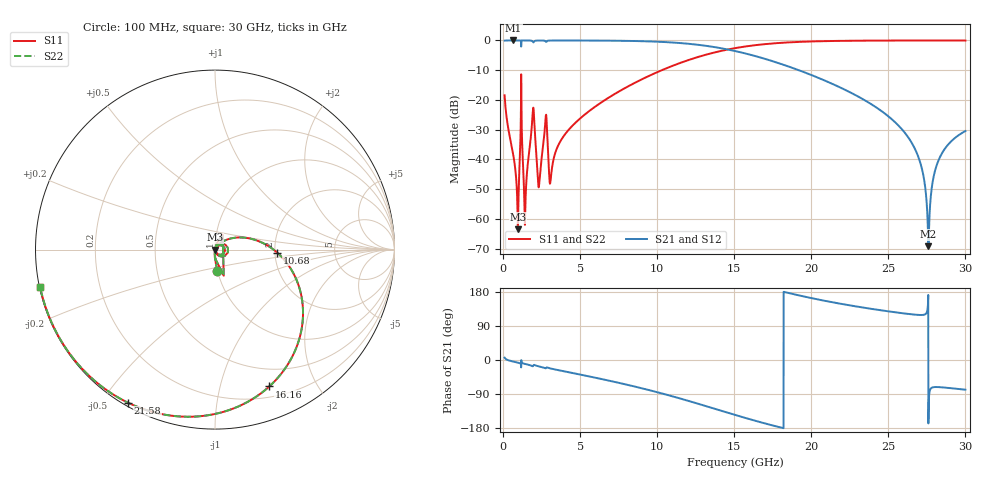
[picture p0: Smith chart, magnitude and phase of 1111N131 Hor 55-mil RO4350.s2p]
# GHz S MA R 50
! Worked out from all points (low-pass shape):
!   3201 points, 100 MHz to 30 GHz, reference 50 ohm
!   highest |S21| = -0.01 dB at 660.6 MHz (marker M1); lowest = -69.2 dB at 27.6 GHz (marker M2)
!   |S21| within 3 dB of the highest: start of sweep to 14.54 GHz
!   lowest |S11| = -63.5 dB at 959.6 MHz (marker M3), VSWR 1.00, Z = 50.1 - j0.0252 ohm
!   |S11| at or under -10 dB: start of sweep to 10.3 GHz
!   |S22| runs from -63.5 to 0.0 dB; largest |S21 - S12| = 0
!   S11 on the Smith chart (normalised r, x): 100 MHz: 1.00, -0.24; 10.68 GHz: 2.06, -0.08; 16.16 GHz: 0.31, -1.43; 21.58 GHz: 0.01, -0.58; 30 GHz: 0.00, -0.10
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0.1  0.1197 -83.7  0.9926 6.1  0.9926 6.1  0.1197 -83.7
0.660625  0.01189 -91.9  0.9994 -4.1  0.9994 -4.1  0.01189 -91.9
0.959625  0.0006712 -22.0  0.9992 -7.0  0.9992 -7.0  0.0006712 -22.0
1.183875  0.1533 -71.5  0.9398 -0.3  0.9398 -0.3  0.1533 -71.5
1.492219  0.003471 63.5  0.9989 -11.0  0.9989 -11.0  0.003471 63.5
1.922031  0.05953 30.9  0.9585 -16.5  0.9585 -16.5  0.05953 30.9
2.333156  0.003607 11.6  0.9966 -17.0  0.9966 -17.0  0.003607 11.6
2.734938  0.04014 35.7  0.9775 -21.7  0.9775 -21.7  0.04014 35.7
3.108687  0.005107 32.5  0.9967 -22.7  0.9967 -22.7  0.005107 32.5
3.697344  0.01972 57.9  0.9979 -27.7  0.9979 -27.7  0.01972 57.9
5.089563  0.05105 49.3  0.9967 -39.1  0.9967 -39.1  0.05105 49.3
10.06978  0.2978 3.9  0.951 -85.7  0.951 -85.7  0.2978 3.9
10.67713  0.3468 -2.8  0.934 -92.3  0.934 -92.3  0.3468 -2.8
15.05  0.742 -55.2  0.6639 -144.9  0.6639 -144.9  0.742 -55.2
16.16191  0.8203 -68.3  0.5645 -158.0  0.5645 -158.0  0.8203 -68.3
20.03956  0.962 -107.3  0.26 163.1  0.26 163.1  0.962 -107.3
21.58128  0.9811 -119.6  0.1757 150.8  0.1757 150.8  0.9811 -119.6
25.01978  0.9956 -142.4  0.0525 128.3  0.0525 128.3  0.9956 -142.4
26.87919  0.9969 -152.7  0.01221 119.2  0.01221 119.2  0.9969 -152.7
27.59866  0.997 -156.5  0.000347 -167.4  0.000347 -167.4  0.997 -156.5
28.29944  0.9969 -160.0  0.01023 -71.6  0.01023 -71.6  0.9969 -160.0
30  0.9965 -168.1  0.02995 -78.4  0.02995 -78.4  0.9965 -168.1
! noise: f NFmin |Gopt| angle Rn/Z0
0.1  0.0006635  0.7337  1.064  0.0004973
3.417  0.01078  0.5172  24.44  0.003742
6.743  0.01515  0.3979  44.53  0.003576
10.06  0.02277  0.4243  61.13  0.005083
13.39  0.03451  0.5097  76.73  0.008018
16.7  0.05602  0.6411  94.16  0.01443
20.03  0.1045  0.7861  113.8  0.03097
23.35  0.2517  0.9049  133.5  0.09156
26.67  1.6  0.984  151.8  1.391
30  0.8815  0.9703  168  0.07611
